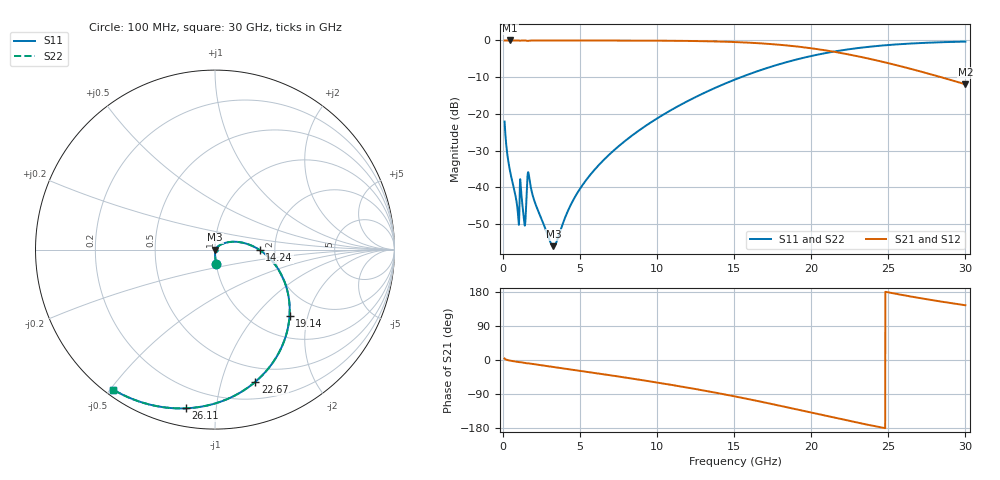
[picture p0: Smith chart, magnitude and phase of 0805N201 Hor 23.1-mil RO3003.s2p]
# GHz S MA R 50
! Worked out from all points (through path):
!   3201 points, 100 MHz to 30 GHz, reference 50 ohm
!   highest |S21| = -0.01 dB at 464.4 MHz (marker M1); lowest = -11.9 dB at 30 GHz (marker M2)
!   group delay of S21, straight-line fit = 20.9 ps
!   lowest |S11| = -56.0 dB at 3.268 GHz (marker M3), VSWR 1.00, Z = 50.1 - j0.0545 ohm
!   |S11| at or under -10 dB: start of sweep to 15.44 GHz
!   |S22| runs from -56.0 to -0.3 dB; largest |S21 - S12| = 0
!   S11 on the Smith chart (normalised r, x): 100 MHz: 1.00, -0.16; 14.24 GHz: 1.67, -0.01; 19.14 GHz: 1.44, -1.55; 22.67 GHz: 0.36, -1.29; 26.11 GHz: 0.09, -0.83; 30 GHz: 0.02, -0.51
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0.1  0.07875 -85.9  0.9967 3.9  0.9967 3.9  0.07875 -85.9
0.4644063  0.01619 -89.9  0.9993 -1.7  0.9993 -1.7  0.01619 -89.9
0.9129063  0.005622 -84.9  0.999 -4.9  0.999 -4.9  0.005622 -84.9
1.202562  0.007432 -77.9  0.9976 -6.4  0.9976 -6.4  0.007432 -77.9
1.361406  0.003485 -60.5  0.9978 -7.6  0.9978 -7.6  0.003485 -60.5
1.4455  0.003417 -13.9  0.9965 -8.2  0.9965 -8.2  0.003417 -13.9
1.623031  0.01611 -34.4  0.9854 -8.8  0.9854 -8.8  0.01611 -34.4
1.707125  0.01325 -65.3  0.9925 -9.0  0.9925 -9.0  0.01325 -65.3
2.136938  0.005688 -82.9  0.9981 -11.8  0.9981 -11.8  0.005688 -82.9
3.267531  0.001587 -20.0  0.9983 -18.4  0.9983 -18.4  0.001587 -20.0
4.332719  0.005462 46.7  0.9981 -24.6  0.9981 -24.6  0.005462 46.7
5.089563  0.01028 50.4  0.9979 -29.1  0.9979 -29.1  0.01028 50.4
7.145187  0.03132 44.4  0.997 -41.4  0.997 -41.4  0.03132 44.4
10.06978  0.08884 28.1  0.9927 -59.9  0.9927 -59.9  0.08884 28.1
14.23709  0.2499 -0.7  0.9635 -89.7  0.9635 -89.7  0.2499 -0.7
15.05  0.2938 -7.0  0.9508 -96.1  0.9508 -96.1  0.2938 -7.0
19.14256  0.5572 -41.8  0.8236 -131.2  0.8236 -131.2  0.5572 -41.8
20.03956  0.6167 -49.9  0.78 -139.3  0.78 -139.3  0.6167 -49.9
22.66516  0.7699 -73.0  0.6301 -162.5  0.6301 -162.5  0.7699 -73.0
25.01978  0.8671 -92.2  0.4893 178.3  0.4893 178.3  0.8671 -92.2
26.113  0.8992 -100.4  0.4285 170.0  0.4285 170.0  0.8992 -100.4
30  0.9645 -125.9  0.2531 144.5  0.2531 144.5  0.9645 -125.9
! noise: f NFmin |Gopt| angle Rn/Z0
0.1  0.0003687  0.8387  0.6373  0.0004837
3.417  0.005639  0.6745  19.26  0.00325
6.743  0.009248  0.6277  37.31  0.004204
10.06  0.01299  0.6186  54.19  0.005101
13.39  0.0172  0.6281  69.84  0.005978
16.7  0.0223  0.6506  84.24  0.006919
20.03  0.02891  0.6837  97.73  0.008021
23.35  0.03795  0.7258  110.6  0.009383
26.67  0.0512  0.7752  123.3  0.01108
30  0.07197  0.828  136  0.01303
